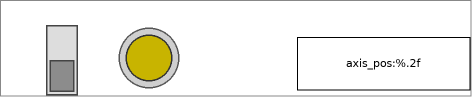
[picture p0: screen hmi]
VISUALIZATION hmi  // 472x97
    DipSwitch (27,25 70x70), variable: MAIN.home_do, behaviour: TOGGLE, style: Switch-DipSwitch-Gray
    Lamp1 (114,23 70x70), variable: MAIN.sensor, style: Lamp-Lamp1-Yellow
    Rectangle (297,37 173x53), "axis_pos:%.2f", text variable: MAIN.el2521_axis.NcToPlc.ActPos
END_VISUALIZATION
